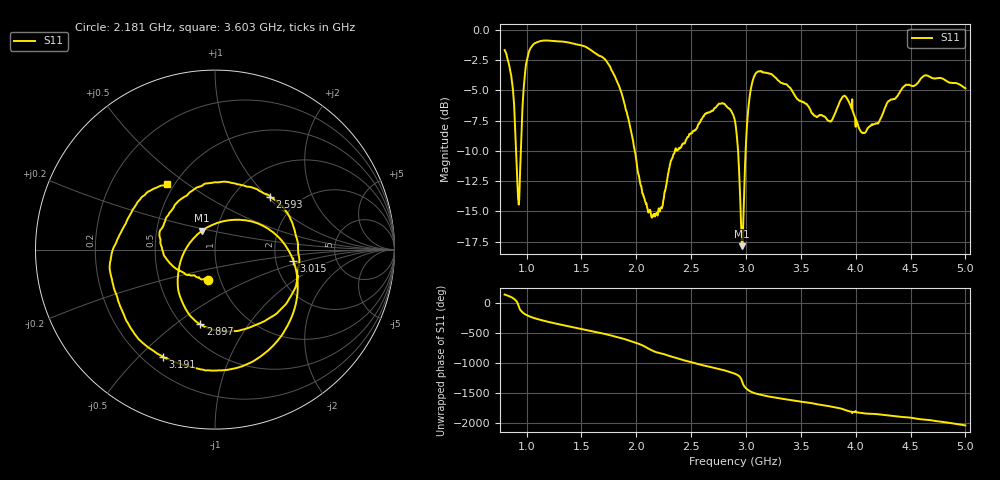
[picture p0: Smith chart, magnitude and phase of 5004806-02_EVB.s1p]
#  HZ  S  RI  R  50.00
! Rohde & Schwarz ZVA/B
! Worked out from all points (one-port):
!   1601 points, 800 MHz to 5 GHz, reference 50 ohm
!   lowest |S11| = -17.9 dB at 2.966 GHz (marker M1), VSWR 1.29, Z = 42.3 + j9.01 ohm
!   |S11| at or under -10 dB: 904.2 MHz to 947.9 MHz (43.61 MHz wide, 4.71 % of centre); 1.986 GHz to 2.352 GHz (365.9 MHz wide, 16.9 % of centre); 2.928 GHz to 2.997 GHz (68.83 MHz wide, 2.32 % of centre)
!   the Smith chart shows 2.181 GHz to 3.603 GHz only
!   S11 on the Smith chart (normalised r, x): 2.181 GHz: 0.88, -0.31; 2.593 GHz: 1.44, +1.04; 2.897 GHz: 0.61, -0.62; 3.015 GHz: 2.51, -0.39; 3.191 GHz: 0.28, -0.59; 3.603 GHz: 0.46, +0.42
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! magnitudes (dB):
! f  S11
! 800 MHz  -1.7
! 868.2 MHz  -4.3
! 926 MHz  -14.1
! 941.8 MHz  -11.6
! 981.1 MHz  -4.1
! 1.02 GHz  -1.9
! 1.325 GHz  -1.0
! 1.7 GHz  -2.3
! 1.85 GHz  -4.8
! 2.068 GHz  -13.7
! 2.181 GHz  -15.2
! 2.375 GHz  -9.9
! 2.593 GHz  -7.4
! 2.784 GHz  -6.1
! 2.897 GHz  -7.5
! 2.9 GHz  -7.5
! 2.966 GHz  -17.9
! 3.015 GHz  -7.1
! 3.076 GHz  -3.8
! 3.191 GHz  -3.6
! 3.425 GHz  -5.1
! 3.603 GHz  -6.9
! 3.766 GHz  -7.6
! 3.884 GHz  -5.5
! 3.95 GHz  -6.2
! 4.076 GHz  -8.5
! 4.475 GHz  -4.6
! 5 GHz  -4.8
